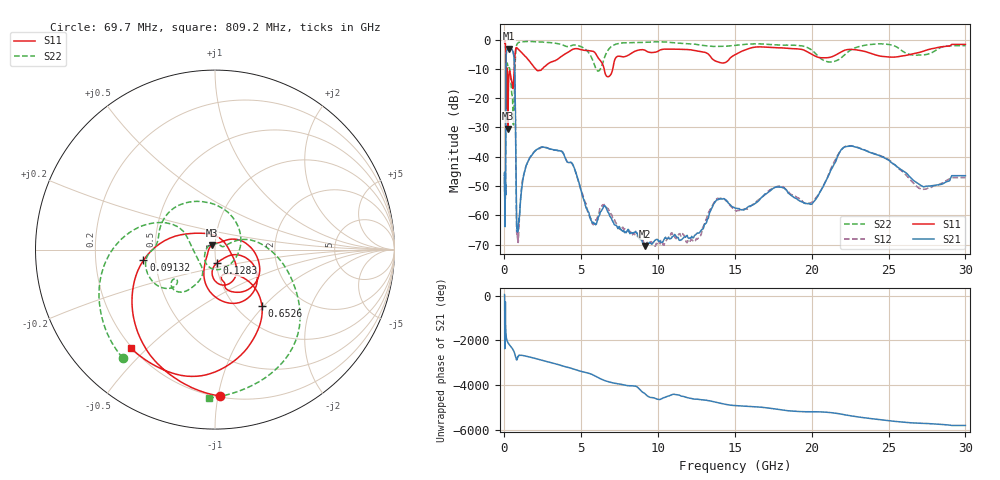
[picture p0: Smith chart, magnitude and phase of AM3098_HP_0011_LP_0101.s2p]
! Date/Time: Thu, Feb 28, 2019 8:34 AM
! Network Analyzer: Agilent Technologies E8364B Rev: A.07.50.67
! Sweep from 0.010 to 30.000 GHz, 1601 Points, Sweep Type: LOG
! Power Supply: 5.022 V, 0.002 A
# Hz S DB R 50
!freq MagS11 AngS11 MagS21 AngS21 MagS12 AngS12 MagS22 AngS22
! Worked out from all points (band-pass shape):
!   1601 points, 10 MHz to 30 GHz, reference 50 ohm
!   highest |S21| = -3.07 dB at 266.5 MHz (marker M1); lowest = -70.5 dB at 9.164 GHz (marker M2)
!   |S21| within 3 dB of the highest: 107.6 MHz to 618.9 MHz (511.2 MHz wide, 141 % of centre)
!   lowest |S11| = -30.4 dB at 228.2 MHz (marker M3), VSWR 1.06, Z = 48.3 + j2.44 ohm
!   |S11| at or under -10 dB: 175.9 MHz to 632 MHz (456.1 MHz wide, 113 % of centre); 2.023 GHz to 2.46 GHz (437.8 MHz wide, 19.5 % of centre); 6.489 GHz to 7.049 GHz (559.6 MHz wide, 8.27 % of centre)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
!   |S22| runs from -29.1 to -0.5 dB; largest |S21 - S12| = 0.0097
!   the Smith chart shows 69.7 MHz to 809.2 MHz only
!   S11 on the Smith chart (normalised r, x): 69.7 MHz: 0.21, -1.02; 91.32 MHz: 0.43, -0.06; 128.3 MHz: 1.01, -0.15; 652.6 MHz: 1.29, -0.98; 809.2 MHz: 0.19, -0.45
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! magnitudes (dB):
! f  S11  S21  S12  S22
! 10 MHz  -0.3  -46.4  -47.5  -0.5
! 38.04 MHz  -0.5  -61.0  -58.5  -0.9
! 69.7 MHz  -1.8  -51.8  -52.0  -2.0
! 77.42 MHz  -2.5  -50.8  -48.7  -2.7
! 91.32 MHz  -7.9  -20.0  -19.8  -9.3
! 100.9 MHz  -23.6  -8.1  -8.1  -17.0
! 128.3 MHz  -22.3  -4.2  -4.2  -11.0
! 144.7 MHz  -14.1  -3.7  -3.6  -10.4
! 185.8 MHz  -11.2  -3.5  -3.5  -8.1
! 228.2 MHz  -30.4  -3.2  -3.1  -9.6
! 266.5 MHz  -14.6  -3.1  -3.0  -9.8
! 550.5 MHz  -16.7  -4.1  -4.1  -24.8
! 652.6 MHz  -7.8  -8.7  -8.7  -17.4
! 809.2 MHz  -2.8  -64.2  -66.4  -1.6
! 2.084 GHz  -10.4  -37.6  -37.7  -0.7
! 3.742 GHz  -5.6  -38.3  -38.2  -1.7
! 6.11 GHz  -6.3  -60.7  -59.9  -10.8
! 7.926 GHz  -5.7  -66.0  -65.1  -1.1
! 9.164 GHz  -3.7  -70.5  -70.5  -0.9
! 19.8 GHz  -4.5  -55.9  -56.0  -2.9
! 22.56 GHz  -3.4  -36.4  -36.3  -3.5
! 30 GHz  -1.7  -46.5  -47.2  -2.1
